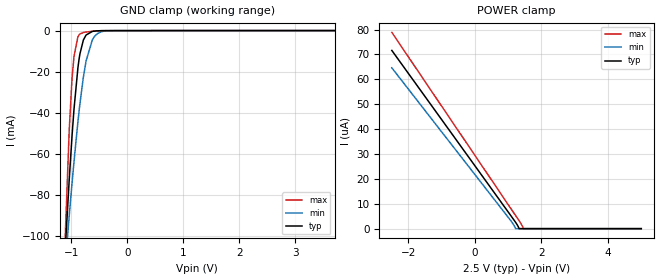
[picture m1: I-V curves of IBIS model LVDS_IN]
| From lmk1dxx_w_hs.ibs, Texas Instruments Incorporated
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|   LVDS_IN Input Model
[Model]   LVDS_IN
Model_type   Input
Vinl = 0.8
Vinh = 1.2
|   typ   min   max
C_comp   3.072pF   2.794pF   3.250pF
[Voltage Range]   2.5   2.375   2.625
[Temperature Range]   45   150   -40
[Power Clamp Reference]   2.5   2.375   2.625
[GND Clamp Reference]   0   0   0
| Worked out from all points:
|   GND clamp passes 1 mA (typ) near -0.66 V on its own axis
[GND Clamp]
|   Voltage   I(typ)   I(min)   I(max)
-2.5V     -947.7mA   -658.1mA   -1.611A
-1.122V   -112.7mA   -118.2mA   -109.5mA
-1.038V   -72.53mA   -90.17mA   -48.59mA
-982.8mV  -49.28mA   -72.73mA   -21.63mA
-952.7mV  -38.26mA   -63.75mA   -12.6mA
-883.8mV  -18.34mA   -44.66mA   -3.158mA
-847.8mV  -11.43mA   -35.77mA   -1.659mA
-784.7mV  -4.546mA   -22.48mA   -935uA
-737.5mV  -2.167mA   -14.78mA   -718.1uA
-625mV    -404.2uA   -4.52mA    -330uA
-439mV    -47.12uA   -399.1uA   -42.76uA
5V        0A         0A         0A
[POWER Clamp]
|   Voltage   I(typ)   I(min)   I(max)
-2.5V     71.64uA    64.65uA    78.88uA
1.06V     5.577uA    3.508uA    8.466uA
1.159V    3.723uA    1.627uA    6.493uA
1.222V    2.545uA    16.73nA    5.261uA
1.326V    9.757nA    0A         3.195uA
1.414V    0A         0A         1.314uA
1.457V    0A         0A         2.627nA
5V        0A         0A         0A
